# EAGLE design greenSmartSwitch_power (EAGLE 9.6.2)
DATABASE: Z:\Eigene Dateien\Anwendungsdaten\Eagle\partdb\exp.txt

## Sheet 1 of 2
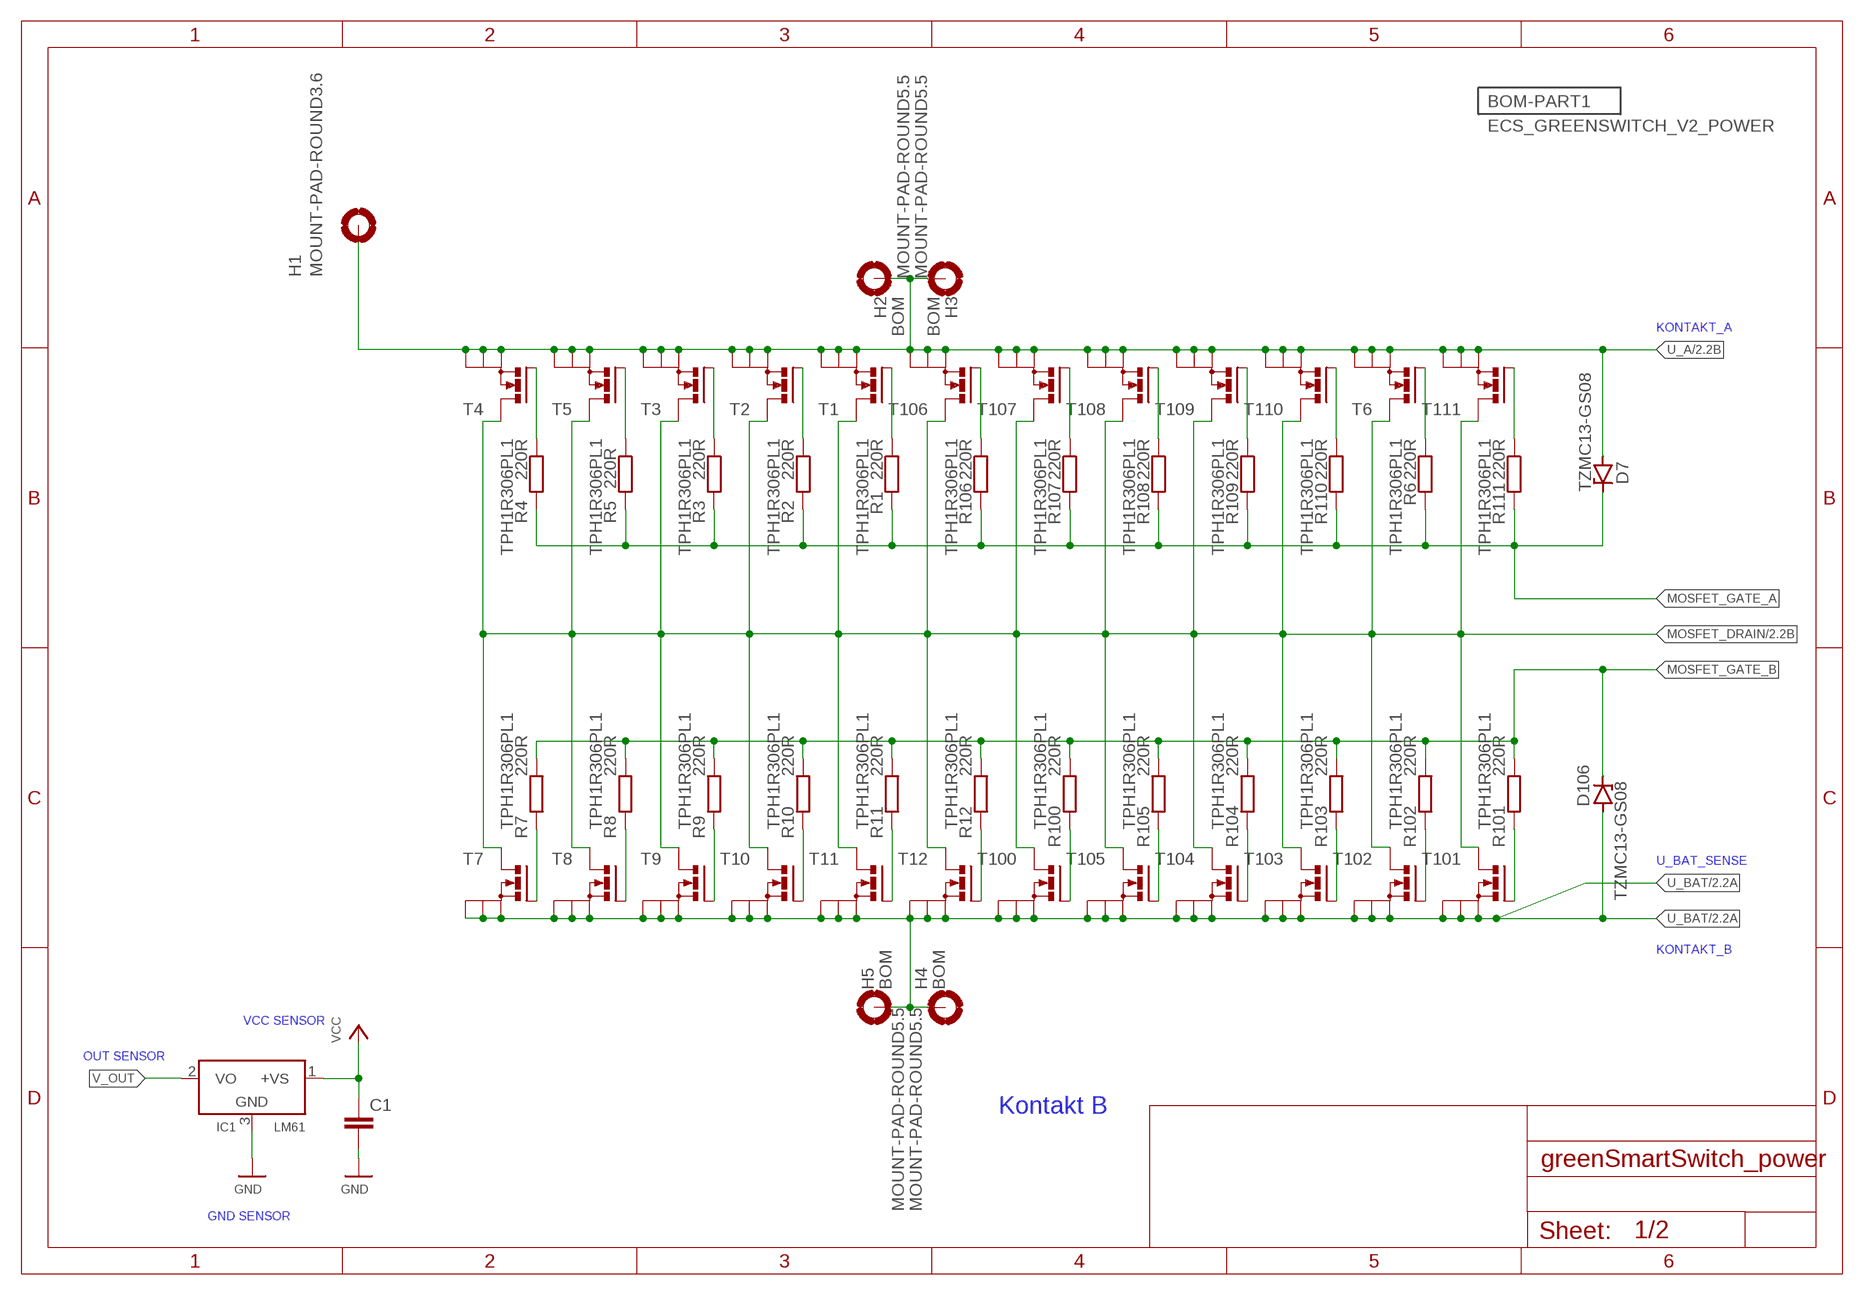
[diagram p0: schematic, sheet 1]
BOM-PART1 (BOM-PART): BOM: INCLUDE; PARTNO: PT067; QTY: 1

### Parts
C1  C-EUC0603  [C0603]
D7  TZMC13-GS08  ZENER-DIODESOD80C  [SOD80C]
D106  TZMC13-GS08  ZENER-DIODESOD80C  [SOD80C]
H1  MOUNT-PAD-ROUND3.6  [3,6-PAD]
H2  MOUNT-PAD-ROUND5.5  [5,5-PAD]
H3  MOUNT-PAD-ROUND5.5  [5,5-PAD]
H4  MOUNT-PAD-ROUND5.5  [5,5-PAD]
H5  MOUNT-PAD-ROUND5.5  [5,5-PAD]
IC1  LM61  LM50  [SOT23]
R1  220R  R-EU_R0603  [R0603]
R2  220R  R-EU_R0603  [R0603]
R3  220R  R-EU_R0603  [R0603]
R4  220R  R-EU_R0603  [R0603]
R5  220R  R-EU_R0603  [R0603]
R6  220R  R-EU_R0603  [R0603]
R7  220R  R-EU_R0603  [R0603]
R8  220R  R-EU_R0603  [R0603]
R9  220R  R-EU_R0603  [R0603]
R10  220R  R-EU_R0603  [R0603]
R11  220R  R-EU_R0603  [R0603]
R12  220R  R-EU_R0603  [R0603]
R100  220R  R-EU_R0603  [R0603]
R101  220R  R-EU_R0603  [R0603]
R102  220R  R-EU_R0603  [R0603]
R103  220R  R-EU_R0603  [R0603]
R104  220R  R-EU_R0603  [R0603]
R105  220R  R-EU_R0603  [R0603]
R106  220R  R-EU_R0603  [R0603]
R107  220R  R-EU_R0603  [R0603]
R108  220R  R-EU_R0603  [R0603]
R109  220R  R-EU_R0603  [R0603]
R110  220R  R-EU_R0603  [R0603]
R111  220R  R-EU_R0603  [R0603]
T1  TPH1R306PL1  SIRA20DP-T1-RE3  [PAWERPAK_SO-8]
T2  TPH1R306PL1  SIRA20DP-T1-RE3  [PAWERPAK_SO-8]
T3  TPH1R306PL1  SIRA20DP-T1-RE3  [PAWERPAK_SO-8]
T4  TPH1R306PL1  SIRA20DP-T1-RE3  [PAWERPAK_SO-8]
T5  TPH1R306PL1  SIRA20DP-T1-RE3  [PAWERPAK_SO-8]
T6  TPH1R306PL1  SIRA20DP-T1-RE3  [PAWERPAK_SO-8]
T7  TPH1R306PL1  SIRA20DP-T1-RE3  [PAWERPAK_SO-8]
T8  TPH1R306PL1  SIRA20DP-T1-RE3  [PAWERPAK_SO-8]
T9  TPH1R306PL1  SIRA20DP-T1-RE3  [PAWERPAK_SO-8]
T10  TPH1R306PL1  SIRA20DP-T1-RE3  [PAWERPAK_SO-8]
T11  TPH1R306PL1  SIRA20DP-T1-RE3  [PAWERPAK_SO-8]
T12  TPH1R306PL1  SIRA20DP-T1-RE3  [PAWERPAK_SO-8]
T100  TPH1R306PL1  SIRA20DP-T1-RE3  [PAWERPAK_SO-8]
T101  TPH1R306PL1  SIRA20DP-T1-RE3  [PAWERPAK_SO-8]
T102  TPH1R306PL1  SIRA20DP-T1-RE3  [PAWERPAK_SO-8]
T103  TPH1R306PL1  SIRA20DP-T1-RE3  [PAWERPAK_SO-8]
T104  TPH1R306PL1  SIRA20DP-T1-RE3  [PAWERPAK_SO-8]
T105  TPH1R306PL1  SIRA20DP-T1-RE3  [PAWERPAK_SO-8]
T106  TPH1R306PL1  SIRA20DP-T1-RE3  [PAWERPAK_SO-8]
T107  TPH1R306PL1  SIRA20DP-T1-RE3  [PAWERPAK_SO-8]
T108  TPH1R306PL1  SIRA20DP-T1-RE3  [PAWERPAK_SO-8]
T109  TPH1R306PL1  SIRA20DP-T1-RE3  [PAWERPAK_SO-8]
T110  TPH1R306PL1  SIRA20DP-T1-RE3  [PAWERPAK_SO-8]
T111  TPH1R306PL1  SIRA20DP-T1-RE3  [PAWERPAK_SO-8]

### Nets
GND: C1.2 IC1.3(GND)
MOSFET_DRAIN: T1.D T2.D T3.D T4.D T5.D T6.D T7.D T8.D T9.D T10.D T11.D T12.D T100.D T101.D T102.D T103.D T104.D T105.D T106.D T107.D T108.D T109.D T110.D T111.D ; also sheet 2
MOSFET_GATE_A: D7.C R1.2 R2.2 R3.2 R4.2 R5.2 R6.2 R106.2 R107.2 R108.2 R109.2 R110.2 R111.2
MOSFET_GATE_B: D106.C R7.2 R8.2 R9.2 R10.2 R11.2 R12.2 R100.2 R101.2 R102.2 R103.2 R104.2 R105.2
N$3: R7.1 T7.G
N$4: R8.1 T8.G
N$5: R9.1 T9.G
N$6: R10.1 T10.G
N$7: R11.1 T11.G
N$8: R12.1 T12.G
N$9: R100.1 T100.G
N$10: R105.1 T105.G
N$11: R104.1 T104.G
N$12: R103.1 T103.G
N$13: R111.1 T111.G
N$14: R102.1 T102.G
N$15: R109.1 T109.G
N$16: R108.1 T108.G
N$17: R107.1 T107.G
N$18: R106.1 T106.G
N$19: R1.1 T1.G
N$20: R2.1 T2.G
N$21: R3.1 T3.G
N$22: R5.1 T5.G
N$23: R4.1 T4.G
N$24: R110.1 T110.G
N$26: R6.1 T6.G
N$27: R101.1 T101.G
U_A: D7.A H1.B3,6(MOUNT) H2.B6,4(MOUNT) H3.B6,4(MOUNT) T1.S@1(S) T1.S@2(S) T1.S@3(S) T2.S@1(S) T2.S@2(S) T2.S@3(S) T3.S@1(S) T3.S@2(S) T3.S@3(S) T4.S@1(S) T4.S@2(S) T4.S@3(S) T5.S@1(S) T5.S@2(S) T5.S@3(S) T6.S@1(S) T6.S@2(S) T6.S@3(S) T106.S@1(S) T106.S@2(S) T106.S@3(S) T107.S@1(S) T107.S@2(S) T107.S@3(S) T108.S@1(S) T108.S@2(S) T108.S@3(S) T109.S@1(S) T109.S@2(S) T109.S@3(S) T110.S@1(S) T110.S@2(S) T110.S@3(S) T111.S@1(S) T111.S@2(S) T111.S@3(S) ; also sheet 2
U_BAT: D106.A H4.B6,4(MOUNT) H5.B6,4(MOUNT) T7.S@1(S) T7.S@2(S) T7.S@3(S) T8.S@1(S) T8.S@2(S) T8.S@3(S) T9.S@1(S) T9.S@2(S) T9.S@3(S) T10.S@1(S) T10.S@2(S) T10.S@3(S) T11.S@1(S) T11.S@2(S) T11.S@3(S) T12.S@1(S) T12.S@2(S) T12.S@3(S) T100.S@1(S) T100.S@2(S) T100.S@3(S) T101.S@1(S) T101.S@2(S) T101.S@3(S) T102.S@1(S) T102.S@2(S) T102.S@3(S) T103.S@1(S) T103.S@2(S) T103.S@3(S) T104.S@1(S) T104.S@2(S) T104.S@3(S) T105.S@1(S) T105.S@2(S) T105.S@3(S) ; also sheet 2
V_OUT: IC1.2(VO)
VCC: C1.1 IC1.1(+VS)

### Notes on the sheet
- KONTAKT_A
- U_BAT_SENSE
- KONTAKT_B
- VCC SENSOR
- OUT SENSOR
- Kontakt B
- GND SENSOR

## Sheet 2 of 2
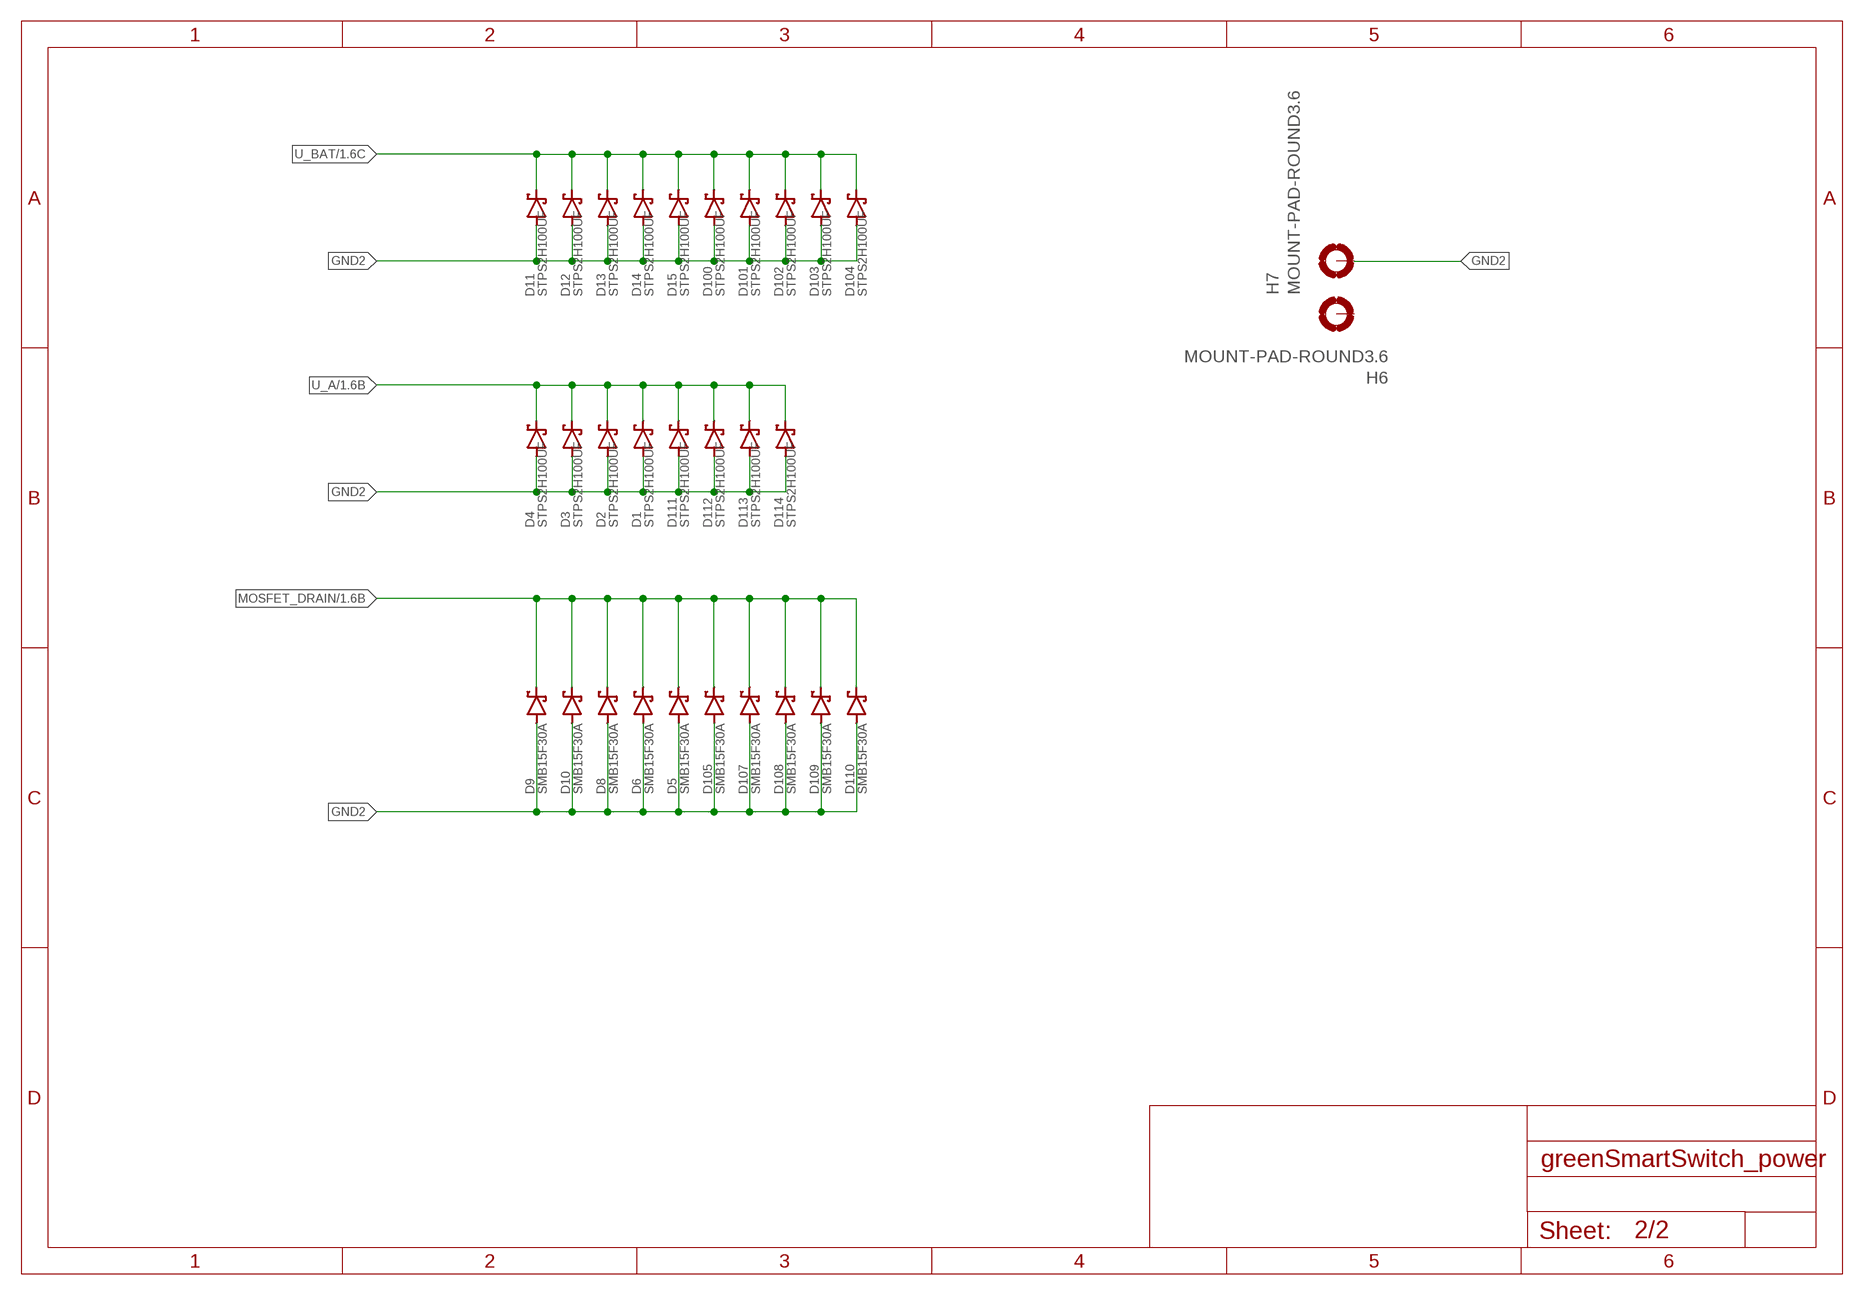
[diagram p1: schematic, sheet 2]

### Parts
D1  STPS2H100UF  SCHOTTKY-DIODESMD  [SMB]
D2  STPS2H100UF  SCHOTTKY-DIODESMD  [SMB]
D3  STPS2H100UF  SCHOTTKY-DIODESMD  [SMB]
D4  STPS2H100UF  SCHOTTKY-DIODESMD  [SMB]
D5  SMB15F30A  SCHOTTKY-DIODESMD  [SMB]
D6  SMB15F30A  SCHOTTKY-DIODESMD  [SMB]
D8  SMB15F30A  SCHOTTKY-DIODESMD  [SMB]
D9  SMB15F30A  SCHOTTKY-DIODESMD  [SMB]
D10  SMB15F30A  SCHOTTKY-DIODESMD  [SMB]
D11  STPS2H100UF  SCHOTTKY-DIODESMD  [SMB]
D12  STPS2H100UF  SCHOTTKY-DIODESMD  [SMB]
D13  STPS2H100UF  SCHOTTKY-DIODESMD  [SMB]
D14  STPS2H100UF  SCHOTTKY-DIODESMD  [SMB]
D15  STPS2H100UF  SCHOTTKY-DIODESMD  [SMB]
D100  STPS2H100UF  SCHOTTKY-DIODESMD  [SMB]
D101  STPS2H100UF  SCHOTTKY-DIODESMD  [SMB]
D102  STPS2H100UF  SCHOTTKY-DIODESMD  [SMB]
D103  STPS2H100UF  SCHOTTKY-DIODESMD  [SMB]
D104  STPS2H100UF  SCHOTTKY-DIODESMD  [SMB]
D105  SMB15F30A  SCHOTTKY-DIODESMD  [SMB]
D107  SMB15F30A  SCHOTTKY-DIODESMD  [SMB]
D108  SMB15F30A  SCHOTTKY-DIODESMD  [SMB]
D109  SMB15F30A  SCHOTTKY-DIODESMD  [SMB]
D110  SMB15F30A  SCHOTTKY-DIODESMD  [SMB]
D111  STPS2H100UF  SCHOTTKY-DIODESMD  [SMB]
D112  STPS2H100UF  SCHOTTKY-DIODESMD  [SMB]
D113  STPS2H100UF  SCHOTTKY-DIODESMD  [SMB]
D114  STPS2H100UF  SCHOTTKY-DIODESMD  [SMB]
H6  MOUNT-PAD-ROUND3.6  [3,6-PAD]
H7  MOUNT-PAD-ROUND3.6  [3,6-PAD]

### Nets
GND2: D1.A D2.A D3.A D4.A D5.A D6.A D8.A D9.A D10.A D11.A D12.A D13.A D14.A D15.A D100.A D101.A D102.A D103.A D104.A D105.A D107.A D108.A D109.A D110.A D111.A D112.A D113.A D114.A H7.B3,6(MOUNT)
MOSFET_DRAIN: D5.C D6.C D8.C D9.C D10.C D105.C D107.C D108.C D109.C D110.C ; also sheet 1
U_A: D1.C D2.C D3.C D4.C D111.C D112.C D113.C D114.C ; also sheet 1
U_BAT: D11.C D12.C D13.C D14.C D15.C D100.C D101.C D102.C D103.C D104.C ; also sheet 1
Unconnected: H6.B3,6(MOUNT)

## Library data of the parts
C1 = rcl:C-EU: CAPACITOR, European symbol; PARTNO: C067; SPICEPREFIX: C
D1-D4 D11-D15 D100-D104 D111-D114 = diode:SCHOTTKY-DIODE: Schottky Diode; PARTNO: D093
D5 D6 D8-D10 D105 D107-D110 = diode:SCHOTTKY-DIODE: Schottky Diode; PARTNO: D211
D7 D106 = diode:ZENER-DIODE: Z-Diode; PARTNO: D022
H1 = holes:MOUNT-PAD-ROUND: MOUNTING PAD, round; PARTNO: *
H2-H5 = holes:MOUNT-PAD-ROUND: MOUNTING PAD, round; BOM: EXCLUDE
H6 H7 = holes:MOUNT-PAD-ROUND: MOUNTING PAD, round; PARTNO: *; SPICEPREFIX: X
IC1 = linear:LM50: SOT-23 Single-Supply Centigrade Temperature Sensor Vout = (10mV/°C x Temp °C) +5mmmV Source: http://cache.national.com/ds/LM/LM50.pdf; PARTNO: IC040
R1-R12 R100-R111 = rcl:R-EU_: RESISTOR, European symbol; PARTNO: R181; SPICEPREFIX: R
T1-T12 T100-T111 = SIRA20DP-T1-RE3 :SIRA20DP-T1-RE3: N-Channel 25 V (D-S) MOSFET; PARTNO: T166

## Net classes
1 PV_IN: clearance 0.4 mm

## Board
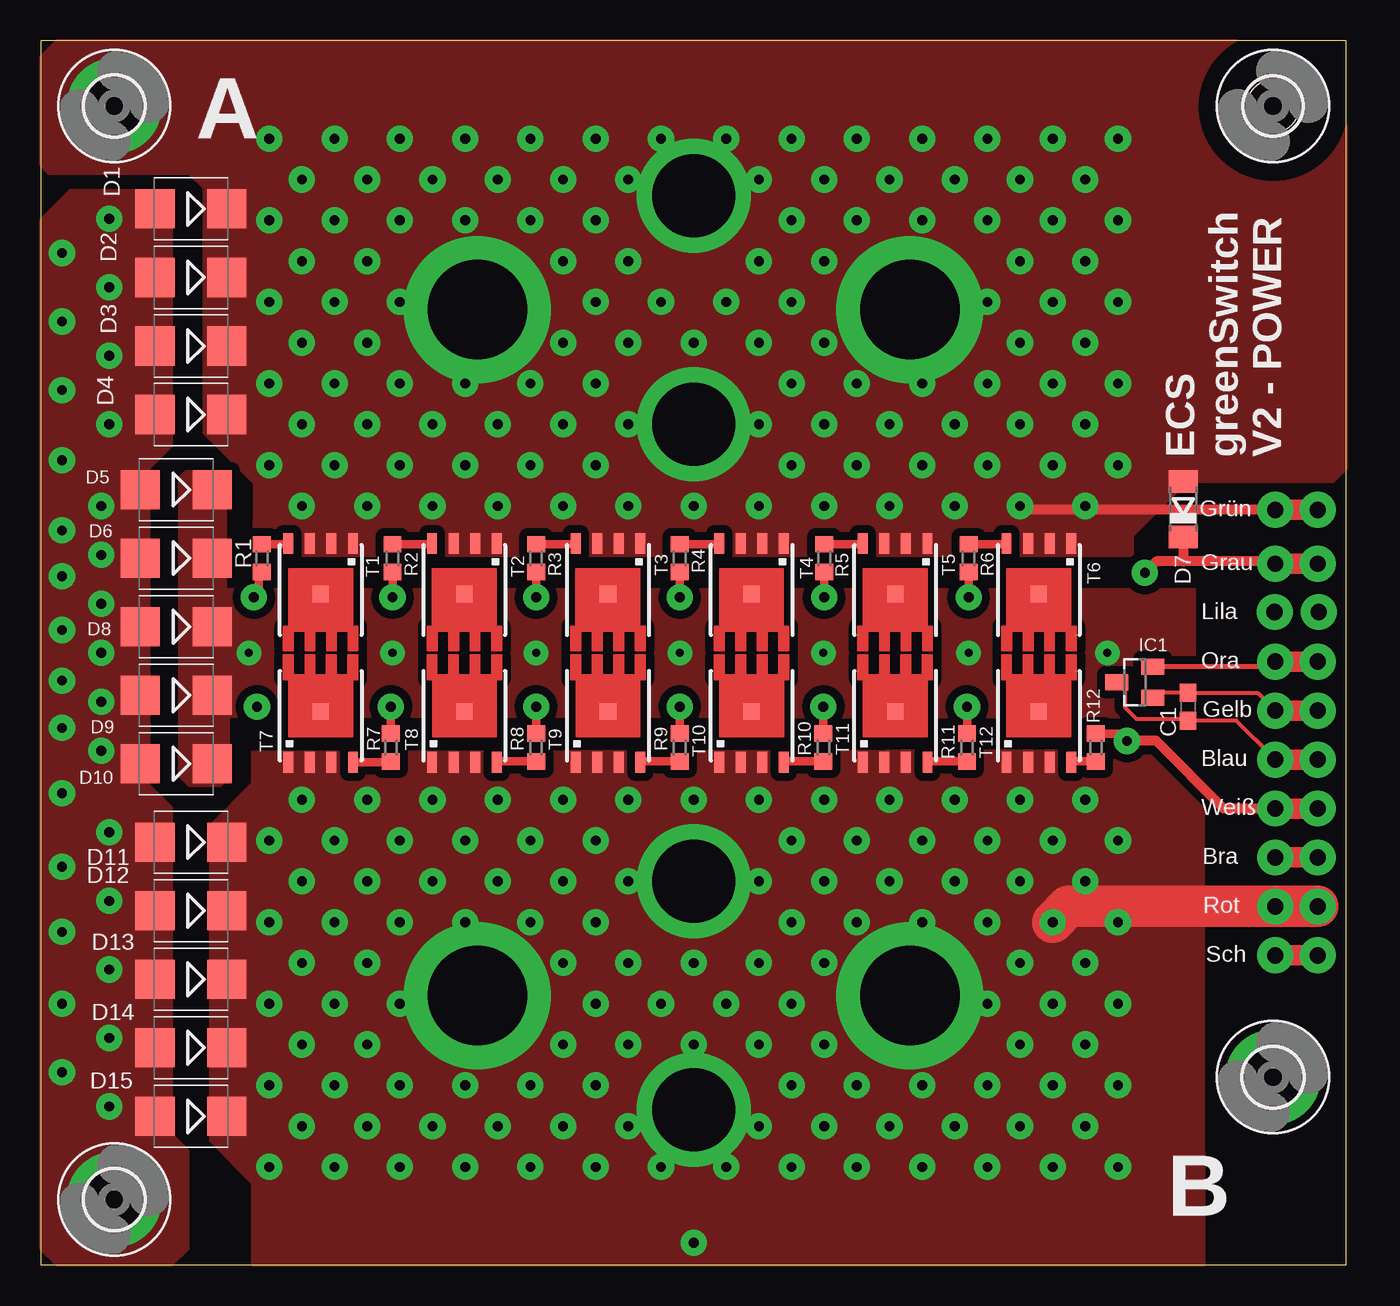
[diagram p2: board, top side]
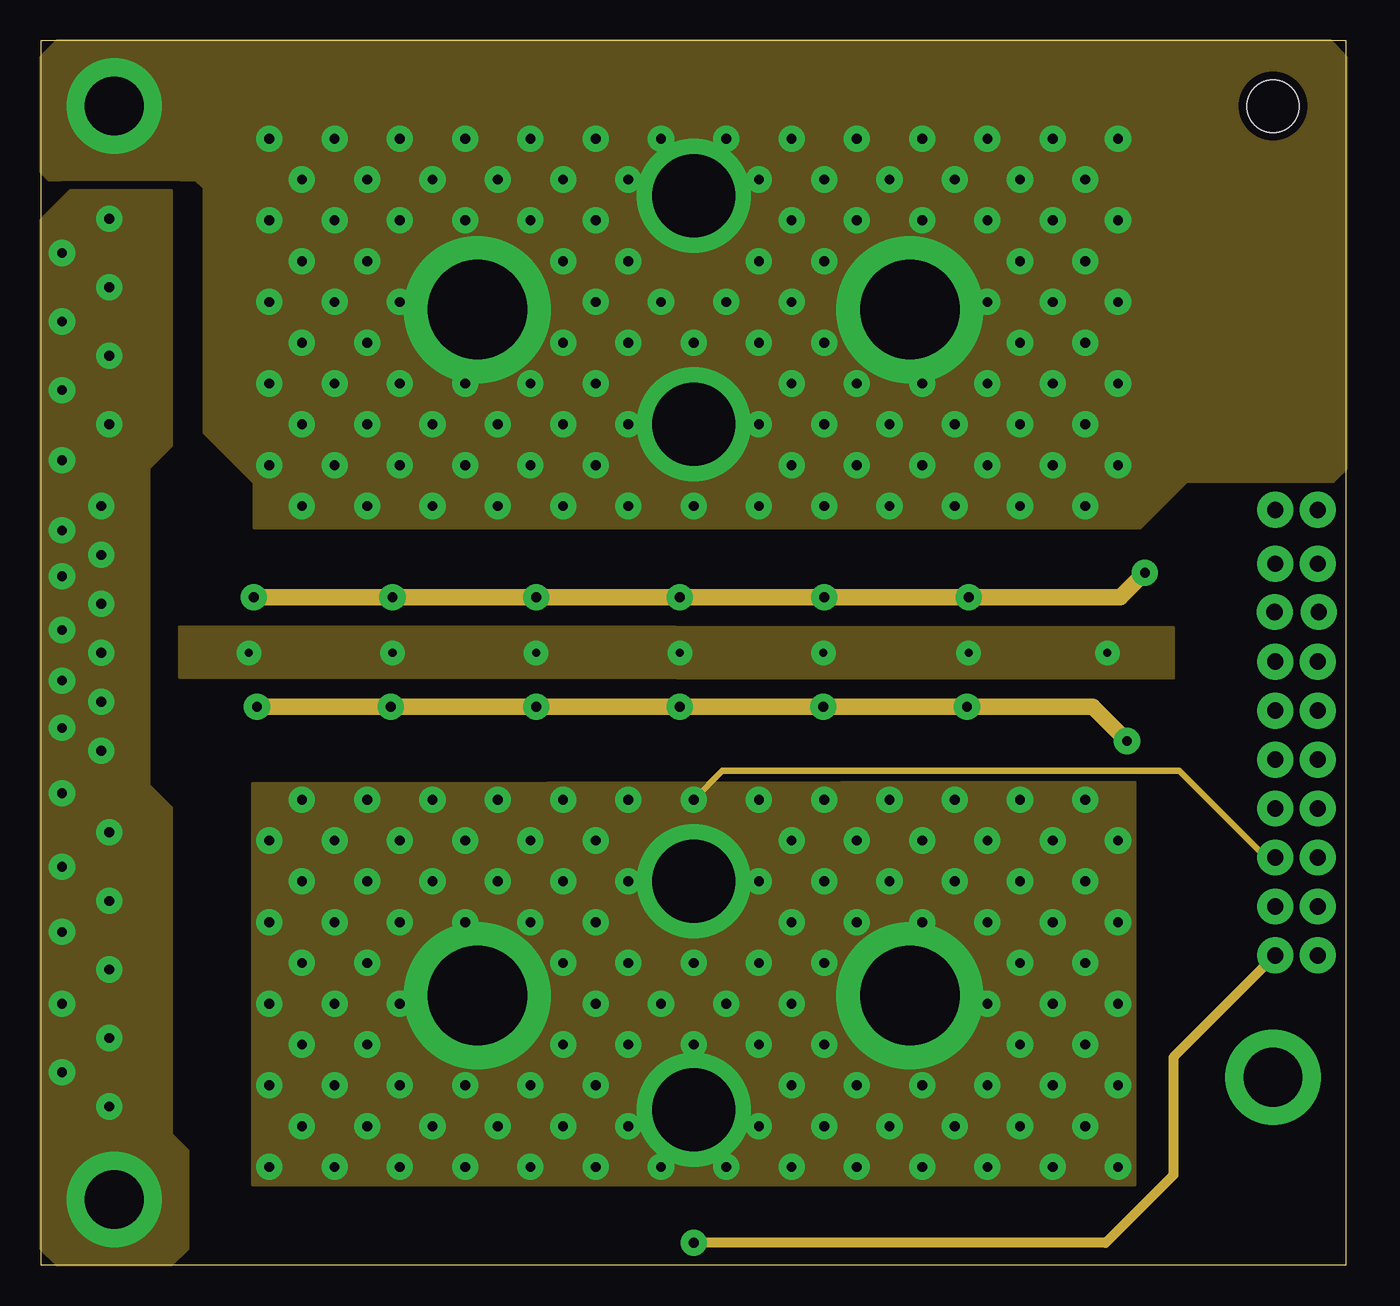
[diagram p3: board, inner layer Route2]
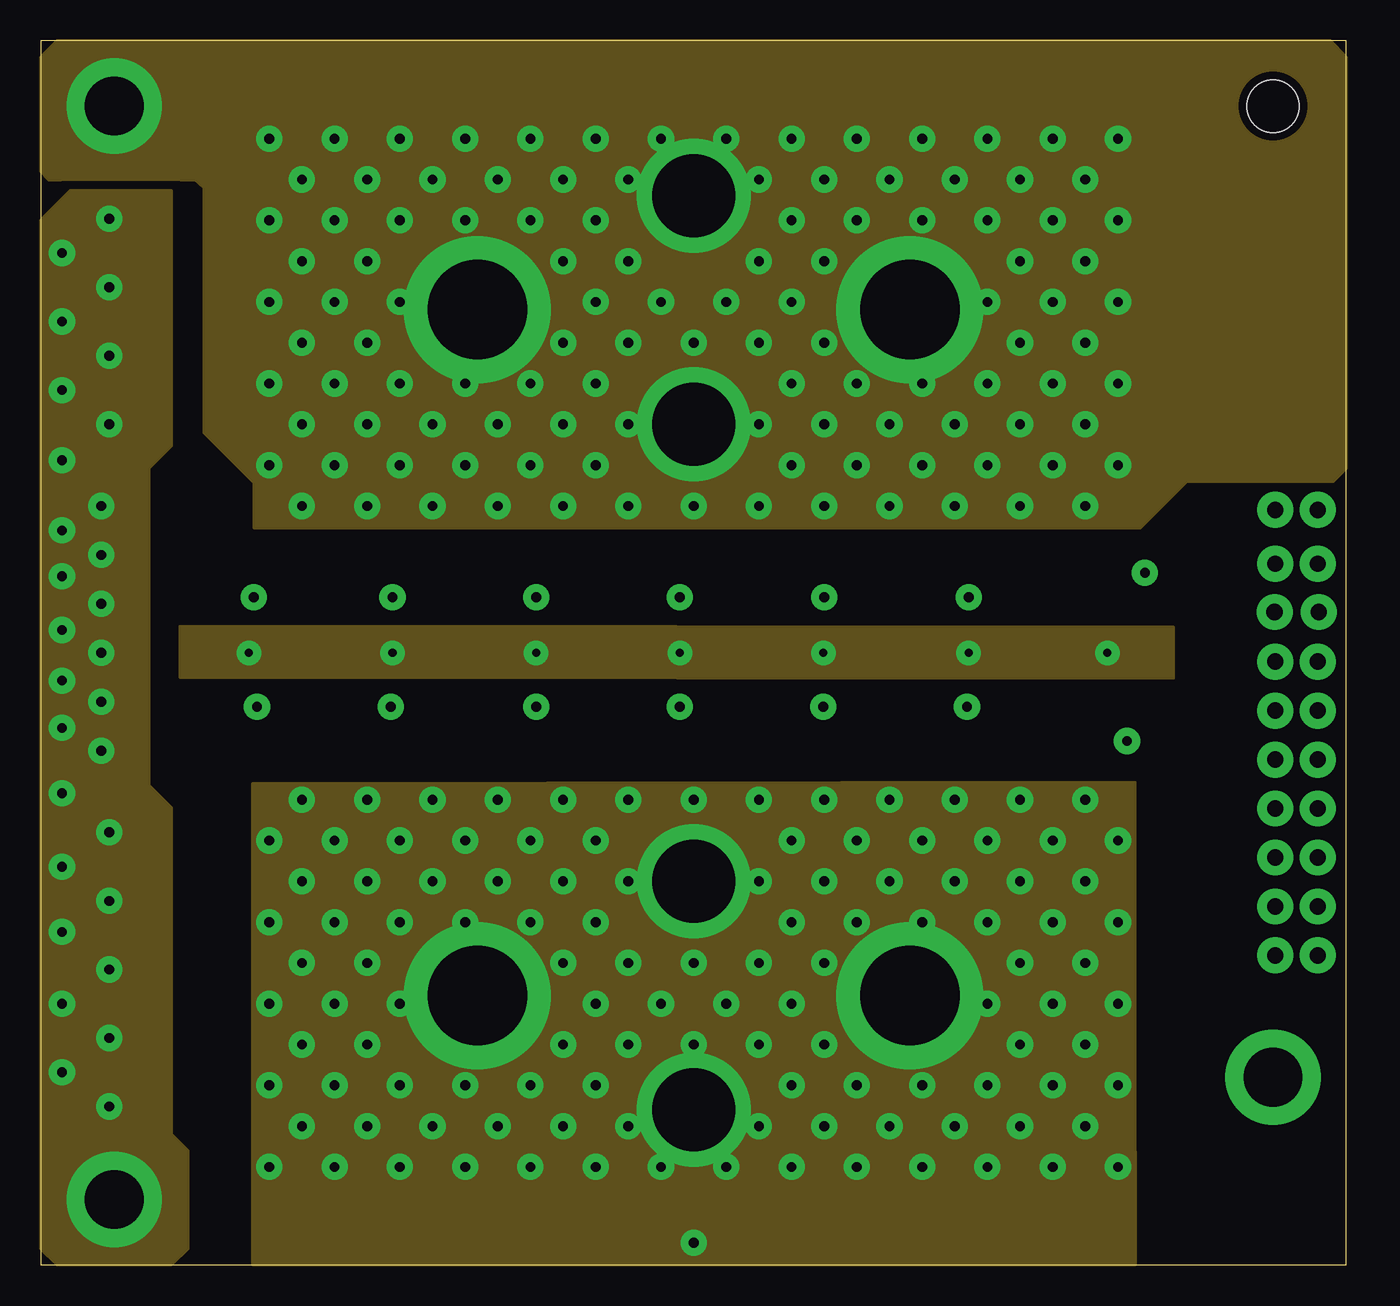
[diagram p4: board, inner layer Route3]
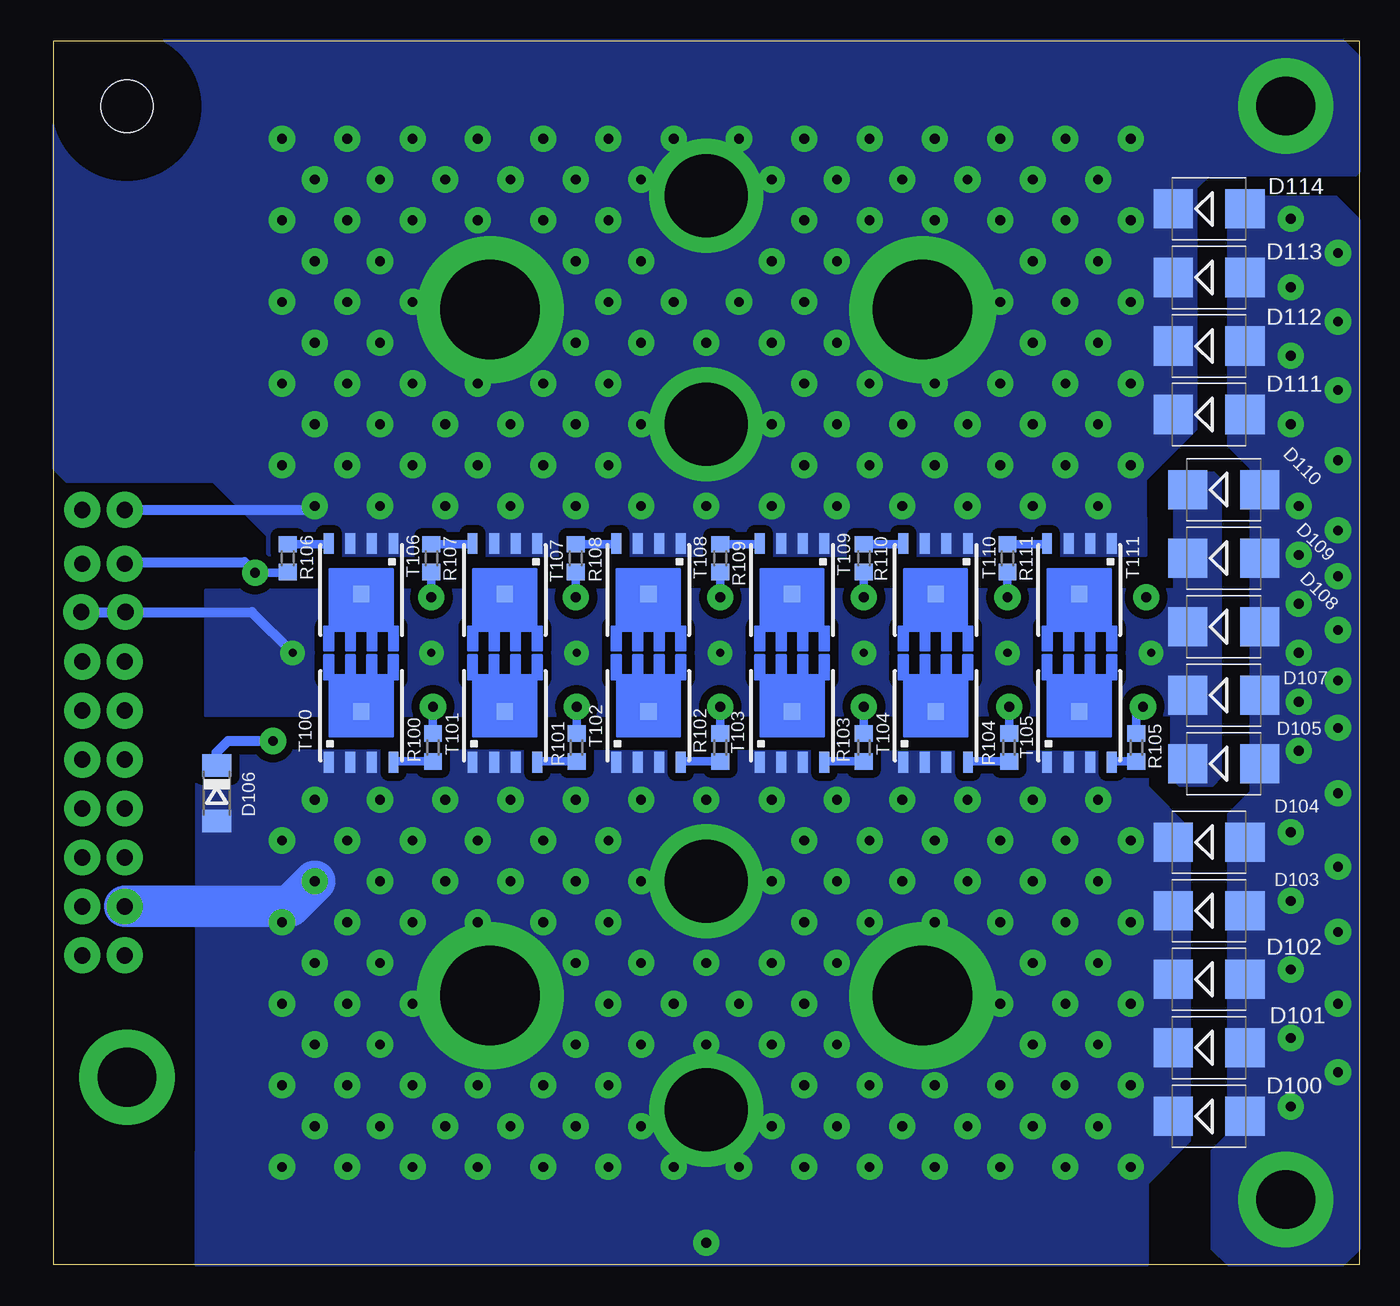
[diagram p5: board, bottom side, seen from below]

Size 80 x 75 mm. Coordinates in mm from the lower left corner, seen from the top.
Outline: 80,0 80,75 0,75 0,0 80,0
Copper layers (1+2*3+16): Top 0.07mm / dielectric 0.3mm / Route2 0.035mm / dielectric 0.75mm / Route3 0.035mm / dielectric 0.3mm / Bottom 0.07mm
Design rules "default *": minimum track width 10mil, minimum drill 0.5mm, track to track 0.5mm, track to pad 0.5mm, pad to pad 0.5mm, via to via 0.5mm, smd to smd 0.15mm, copper to edge 0mil, drill to drill 8mil, minimum pad ring 0.5mm, minimum via ring 0.5mm, stop-mask expansion 4mil, vias tented up to drill 0mil, thermal gap 10mil

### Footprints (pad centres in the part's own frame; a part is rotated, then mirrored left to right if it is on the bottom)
C0603 = smd 1.1 x 1: 1 -0.85,0; 2 0.85,0
SMB = smd 2.4 x 2.4: A 2.2,0; C -2.2,0
SOD80C = smd 1.4 x 1.8: A 1.7,0; C -1.7,0
3,6-PAD = drill 3.6 pad 5.842: B3,6 0,0
5,5-PAD = drill 6.1 pad 9: B6,4 0,0
SOT23 = smd 1 x 1.4: 1 -0.95,-1.1; 2 0.95,-1.1; 3 0,1.1
R0603 = smd 1 x 1.1: 1 -0.85,0; 2 0.85,0
PAWERPAK_SO-8 = smd 1 x 1: D 0,0 | smd 1.27 x 0.61: G -3.1,-1.98; S@1 -3.1,1.98; S@2 -3.1,0.66; S@3 -3.1,-0.66
3,2 = hole 3.2: 0,0

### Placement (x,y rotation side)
C1  70.3,34.2 270 top
D1  9.2,64.7 180 top
D2  9.2,60.5 180 top
D3  9.2,56.3 180 top
D4  9.2,52.1 180 top
D5  8.3,47.5 180 top
D6  8.3,43.3 180 top
D7  70,46.3 90 top
D8  8.3,39.1 180 top
D9  8.3,34.9 180 top
D10  8.3,30.7 180 top
D11  9.2,25.9 180 top
D12  9.2,21.7 180 top
D13  9.2,17.5 180 top
D14  9.2,13.3 180 top
D15  9.2,9.1 180 top
D100  9.2,9.1 0 bottom
D101  9.2,13.3 0 bottom
D102  9.2,17.5 0 bottom
D103  9.2,21.7 0 bottom
D104  9.2,25.9 0 bottom
D105  8.3,30.7 0 bottom
D106  70,28.9 270 bottom
D107  8.3,34.9 0 bottom
D108  8.3,39.1 0 bottom
D109  8.3,43.3 0 bottom
D110  8.3,47.5 0 bottom
D111  9.2,52.1 0 bottom
D112  9.2,56.3 0 bottom
D113  9.2,60.5 0 bottom
D114  9.2,64.7 0 bottom
H1  4.5,71 0 top
H2  26.75,58.52 0 top
H3  53.25,58.52 0 top
H4  26.75,16.5 0 top
H5  53.25,16.5 0 top
H6  75.5,11.5 0 top
H7  4.5,4 0 top
IC1  67.03,35.7 90 top
R1  13.55,43.3 270 top
R2  21.55,43.3 270 top
R3  30.35,43.3 270 top
R4  39.15,43.3 270 top
R5  48,43.3 270 top
R6  56.85,43.3 270 top
R7  21.45,31.7 90 top
R8  30.35,31.7 90 top
R9  39.15,31.7 90 top
R10  47.95,31.7 90 top
R11  56.75,31.7 90 top
R12  64.65,31.7 90 top
R100  56.75,31.7 90 bottom
R101  47.95,31.7 90 bottom
R102  39.15,31.7 90 bottom
R103  30.35,31.7 90 bottom
R104  21.45,31.7 90 bottom
R105  13.65,31.7 90 bottom
R106  65.65,43.3 270 bottom
R107  56.85,43.3 270 bottom
R108  48,43.3 270 bottom
R109  39.15,43.3 270 bottom
R110  30.35,43.3 270 bottom
R111  21.55,43.3 270 bottom
T1  17.15,41.1 270 top
T2  25.95,41.1 270 top
T3  34.75,41.1 270 top
T4  43.55,41.1 270 top
T5  52.35,41.1 270 top
T6  61.15,41.1 270 top
T7  17.15,33.9 90 top
T8  25.95,33.9 90 top
T9  34.75,33.9 90 top
T10  43.55,33.9 90 top
T11  52.35,33.9 90 top
T12  61.15,33.9 90 top
T100  61.15,33.9 90 bottom
T101  52.35,33.9 90 bottom
T102  43.55,33.9 90 bottom
T103  34.75,33.9 90 bottom
T104  25.95,33.9 90 bottom
T105  17.15,33.9 90 bottom
T106  61.15,41.1 270 bottom
T107  52.35,41.1 270 bottom
T108  43.55,41.1 270 bottom
T109  34.75,41.1 270 bottom
T110  25.95,41.1 270 bottom
T111  17.15,41.1 270 bottom
U$3  [3,2]  75.5,71 0 top

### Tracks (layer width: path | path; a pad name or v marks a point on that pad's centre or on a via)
GND  (via drill 1 pad 2.2)
  Top 0.254: IC1.3 66.43,35.2 66.43,34.17 67.16,33.44 70.21,33.44 C1.2 73.25,33.35 75.5,31.1
  Top 0.305: v75.64,30.96 75.5,31.1
  Top 1.27: v78.24,30.96 v75.64,30.96
GND2  (via drill 0.6)
  other vias: 4.2,64.1 4.2,59.9 4.2,55.7 4.2,51.5 3.7,46.5 3.7,43.5 3.7,40.5 3.7,37.5 3.7,34.5 3.7,31.5 4.2,26.5 4.2,22.3 4.2,18.1 4.2,13.9 4.2,9.7 1.3,62 1.3,57.8 1.3,53.6 1.3,49.3 1.3,45 1.3,42.2 1.3,38.9 1.3,35.8 1.3,32.9 1.3,28.9 1.3,24.4 1.3,20.4 1.3,16 1.3,11.8
  pour Top (no thermals): 1,0 0,1 0,64 1.8,65.8 8,65.8 8,50.2 6.6,48.8 6.6,29.4 8,28 8,8 9,7 9,1 8,0
  pour Route2 (no thermals): 1,0 0,1 0,64 1.8,65.8 8,65.8 8,50.2 6.6,48.8 6.6,29.4 8,28 8,8 9,7 9,1 8,0
  pour Route3 (no thermals): 1,0 0,1 0,64 1.8,65.8 8,65.8 8,50.2 6.6,48.8 6.6,29.4 8,28 8,8 9,7 9,1 8,0
  pour Bottom (no thermals): 1,0 0,1 0,64 1.4,65.4 8,65.4 8,50.2 6.6,48.8 6.6,29 8,27.6 8,8 9,7 9,1 8,0
MOSFET_DRAIN  (via drill 0.5, 1 pad 2.2)
  Bottom 0.61: v78.3,40 v75.6,40 67.85,40 v65.35,37.5
  other vias: 47.95,37.5 39.15,37.5 30.35,37.5 21.55,37.5 12.75,37.5 56.85,37.5
  pour Top (isolate 0.5, no thermals): 8.5,29.97 8.5,48.23 8.91,48.6 11,48.6 11.3,48.3 11.3,41.4 70.67,41.38 70.67,33.55 11.5,33.6 11.5,29.9 11,29.4 9.1,29.4
  pour Bottom (isolate 0.5, no thermals): 70.67,41.35 70.67,33.65 11.5,33.7 11.5,29.9 11,29.4 9,29.4 8.5,29.9 8.5,48.1 8.9,48.5 10.9,48.5 11.3,48.1 11.3,41.4
  pour Route2 (isolate 0.5, no thermals): 69.38,39.05 69.38,35.95 8.5,36 8.5,39.1
  pour Route3 (isolate 0.5, no thermals): 8.55,39.13 69.38,39.08 69.38,35.95 8.55,36
MOSFET_GATE_A  (via drill 0.6, 1 pad 2.2)
  Top 0.508: R1.2 13.35,42.25 13.35,41.2 v13.05,40.9 | R111.2 v21.55,40.9 | R110.2 v30.35,40.9 | R109.2 v39.15,40.9 | R108.2 v48,40.9 | R6.2 v56.85,40.9
  Top 0.61: v67.65,42.4 68.35,43.1 70,43.1 | D7.C 70,43.1 | v75.64,42.96 75.64,43.1 70,43.1
  Top 1.27: v78.24,42.96 v75.64,42.96
  Route2 1.016: v13.05,40.9 v21.55,40.9 v30.35,40.9 v39.15,40.9 v48,40.9 v56.85,40.9 66.15,40.9 v67.65,42.4
  Bottom 0.508: v21.55,40.9 R111.2 | v30.35,40.9 R110.2 | v39.15,40.9 R109.2 | v48,40.9 R108.2 | v56.85,40.9 R6.2 | v67.65,42.4 65.7,42.4 R106.2
  Bottom 0.61: v75.64,42.96 75.54,43.06 68.31,43.06 v67.65,42.4
MOSFET_GATE_B  (via drill 0.6, 1 pad 2.2)
  Top 0.508: v66.55,32.1 66.1,32.55 R12.2 | R100.2 v56.75,34.2 | R101.2 v47.95,34.2 | R102.2 v39.15,34.2 | R103.2 v30.35,34.2 | R104.2 v21.45,34.2
  Top 0.61: v75.64,27.96 72.49,27.96 68.35,32.1 v66.55,32.1
  Top 1.27: v78.24,27.96 v75.64,27.96
  Route2 1.016: v13.25,34.2 v21.45,34.2 v30.35,34.2 v39.15,34.2 v47.95,34.2 v56.75,34.2 64.45,34.2 v66.55,32.1
  Bottom 0.508: R100.2 v56.75,34.2 | R101.2 v47.95,34.2 | R102.2 v39.15,34.2 | R103.2 v30.35,34.2 | R104.2 v21.45,34.2 | v13.25,34.2 13.65,33.8 R105.2
  Bottom 0.61: v66.55,32.1 69.3,32.1 70,31.4 D106.C
N$3
  Top 0.508: R7.1 21.4,30.8 T7.G
N$4
  Top 0.508: R8.1 27.98,30.85 T8.G
N$5
  Top 0.508: R9.1 36.78,30.85 T9.G
N$6
  Top 0.508: R10.1 45.58,30.85 T10.G
N$7
  Top 0.508: R11.1 54.38,30.85 T11.G
N$8
  Top 0.508: R12.1 63.18,30.85 T12.G
N$9
  Bottom 0.508: R100.1 59.12,30.85 T100.G
N$10
  Bottom 0.508: R105.1 15.12,30.85 T105.G
N$11
  Bottom 0.508: R104.1 23.92,30.85 T104.G
N$12
  Bottom 0.508: R103.1 32.72,30.85 T103.G
N$13
  Bottom 0.508: R111.1 19.18,44.15 T111.G
N$14
  Bottom 0.508: R102.1 41.52,30.85 T102.G
N$15
  Bottom 0.508: R109.1 36.78,44.15 T109.G
N$16
  Bottom 0.508: R108.1 45.58,44.15 T108.G
N$17
  Bottom 0.508: R107.1 54.38,44.15 T107.G
N$18
  Bottom 0.508: R106.1 63.18,44.15 T106.G
N$19
  Top 0.508: R1.1 15.12,44.15 T1.G
N$20
  Top 0.508: R2.1 23.92,44.15 T2.G
N$21
  Top 0.508: R3.1 32.72,44.15 T3.G
N$22
  Top 0.508: R5.1 50.32,44.15 T5.G
N$23
  Top 0.508: R4.1 41.52,44.15 T4.G
N$24
  Bottom 0.508: R110.1 27.98,44.15 T110.G
N$26
  Top 0.508: R6.1 59.12,44.15 T6.G
N$27
  Bottom 0.508: R101.1 50.32,30.85 T101.G
U_A  (via drill 0.6 pad 0.6, 1 pad 2.2, 5.1 pad 7)
  Top 0.61: v75.64,46.26 60.24,46.26 v60,46.5
  Top 1.27: v78.24,46.26 v75.64,46.26
  Bottom 0.61: v75.64,46.26 64.24,46.26 v64,46.5
  other vias: 40,51.5 40,65.5 20,46.5 24,46.5 28,46.5 32,46.5 36,46.5 40,46.5 44,46.5 48,46.5 52,46.5 56,46.5 62,49 58,49 54,49 50,49 46,49 34,49 30,49 26,49 22,49 18,49 16,46.5 16,51.5 20,51.5 24,51.5 28,51.5 32,51.5 48,51.5 52,51.5 56,51.5 60,51.5 64,51.5 62,54 58,54 50,54 46,54 34,54 30,54 22,54 18,54 16,56.5 20,56.5 32,56.5 36,56.5 40,56.5 44,56.5 48,56.5 60,56.5 64,56.5 62,59 46,59 42,59 38,59 34,59 18,59 44,51.5 36,51.5 54,54 26,54 22,59 58,59 66,54 66,59 66,49 14,49 14,54 14,59 14,64 18,64 22,64 26,64 30,64 34,64 46,64 50,64 54,64 58,64 62,64 66,64 64,61.5 60,61.5 48,61.5 44,61.5 36,61.5 32,61.5 20,61.5 16,61.5 16,66.5 20,66.5 24,66.5 28,66.5 32,66.5 36,66.5 48,66.5 44,66.5 52,66.5 56,66.5 60,66.5 64,66.5 66,69 62,69 58,69 54,69 50,69 46,69 42,69 38,69 34,69 30,69 26,69 22,69 18,69 14,69
  pour Route3 (isolate 0.5, rank 2, no thermals): 13.07,45.17 13.09,47.91 10,51 10,66 9.47,66.5 0.5,66.5 0,67 0,74 1,75 79,75 80,74 80,48.8 79.2,48 70.21,48 67.38,45.17
  pour Route2 (isolate 0.5, rank 2, no thermals): 13.07,45.17 13.09,47.91 10,51 10,66 9.5,66.5 0.5,66.5 0,67 0,74 1,75 79,75 80,74 80,48.8 79.2,48 70.21,48 67.38,45.17
  pour Bottom (isolate 0.5, rank 2, no thermals): 13.08,43.47 13.1,48.1 10,51.2 10,66 9.2,66.8 0.2,66.8 0,67 0,74 1,75 79,75 80,74 80,48.8 79.2,48 70.2,48 66.87,44.67 66.86,43.47
  pour Top (isolate 0.5, rank 2, no thermals): 13.08,43.47 13.1,47.9 10,51 10,66 9.1,66.9 0.5,66.9 0,67.4 0,74 1,75 79,75 80,74 80,48.8 79.2,48 70.2,48 66.87,44.67 66.86,43.47
U_BAT  (via drill 0.6 pad 0.6, 1 pad 2.2, 5.1 pad 7)
  Top 1.27: v78.24,18.96 v75.64,18.96 | v78.24,24.96 v75.64,24.96
  Top 2.54: v78.24,21.96 v75.64,21.96 62.96,21.96 v62,21
  Route2 0.406: v75.64,24.96 75.04,24.96 69.74,30.26 41.76,30.26 v40,28.5
  Route2 0.61: v40,1.35 65.25,1.35 69.4,5.5 69.4,12.72 v75.64,18.96
  Bottom 2.54: v75.64,21.96 65.54,21.96 v64,23.5
  other vias: 40,23.5 40,9.5 64,28.5 62,26 60,28.5 58,26 56,28.5 54,26 52,28.5 50,26 48,28.5 46,26 44,28.5 36,28.5 34,26 32,28.5 30,26 28,28.5 26,26 24,28.5 22,26 20,28.5 18,26 16,28.5 16,23.5 18,21 20,23.5 16,18.5 20,18.5 18,16 24,23.5 28,23.5 32,23.5 48,23.5 52,23.5 56,23.5 60,23.5 22,21 34,21 46,21 58,21 64,18.5 60,18.5 48,18.5 44,18.5 40,18.5 36,18.5 32,18.5 34,16 38,16 42,16 46,16 62,16 30,21 50,21 26,21 44,23.5 36,23.5 54,21 58,16 22,16 66,26 14,26 14,21 66,21 14,16 66,16 16,13.5 20,13.5 32,13.5 36,13.5 40,13.5 44,13.5 48,13.5 60,13.5 64,13.5 66,11 62,11 58,11 54,11 50,11 46,11 34,11 30,11 26,11 22,11 18,11 14,11 16,8.5 20,8.5 24,8.5 28,8.5 32,8.5 36,8.5 44,8.5 48,8.5 52,8.5 56,8.5 60,8.5 64,8.5 66,6 62,6 58,6 54,6 50,6 46,6 42,6 38,6 34,6 30,6 26,6 22,6 18,6 14,6
  pour Top (isolate 0.305, rank 2, no thermals): 13,31.42 13,29.5 10.4,26.9 10.4,7.6 13,5 13,0 71.25,0 71.22,13.93 71.22,31.51
  pour Route3 (isolate 0.305, rank 2, no thermals): 13,29.49 13,0.01 67.05,0.01 67.03,13.94 67.03,29.58
  pour Route2 (isolate 0.305, rank 2, no thermals): 12.99,29.49 12.99,4.9 67.03,4.9 67.02,13.98 67.02,29.58
  pour Bottom (isolate 0.305, rank 2, no thermals): 13,31.42 13,29.3 10.4,26.7 10.4,7.6 13,5 13,0 71.25,0 71.22,13.93 71.22,31.51
V_OUT  (via drill 1 pad 2.2)
  Top 0.305: IC1.2 75.33,36.65 v75.64,36.96
  Top 1.27: v78.24,36.96 v75.64,36.96
VCC  (via drill 1 pad 2.2)
  Top 0.254: IC1.1 68.43,35.05 C1.1 74.55,35.05 v75.64,33.96
  Top 1.27: v78.24,33.96 v75.64,33.96

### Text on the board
tPlace: A | ECS / greenSwitch / V2 - POWER | Grün | Grau | Lila | Ora | Gelb | Blau | Weiß | Bra | Rot | Sch | B
DrillLegend_01-16: 01-16
DrillLegend_01-20: 01-20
